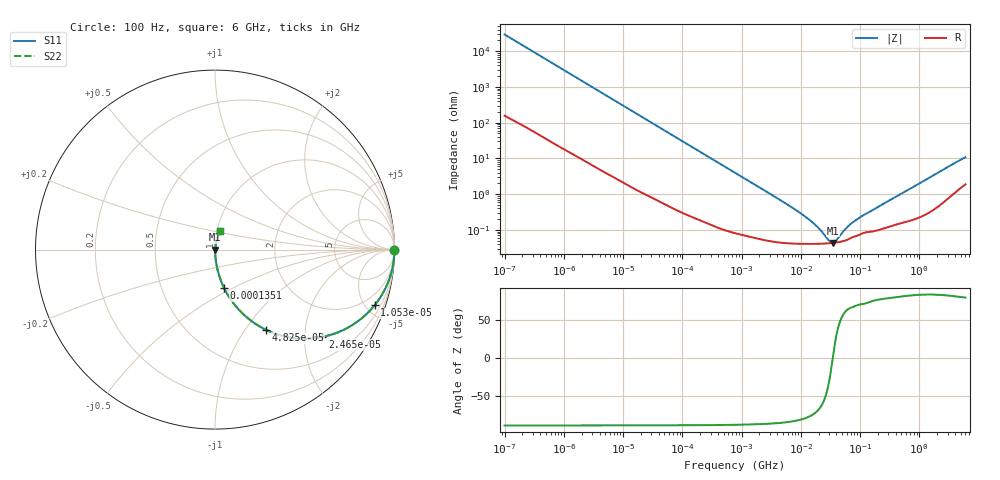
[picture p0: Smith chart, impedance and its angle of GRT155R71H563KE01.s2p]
!Murata Part Number: GRT155R71H563KE01
!These Parameters are Measured in Series Mode Connection
!Data Generated on Jun 19, 2026
!  o--ll--o
!Port1  Port2
!  o------o
!Operation Temp=25[degC], DC Bias Voltage=0[V]
!Freq. Start=100[Hz] Stop=6[GHz] 401[Steps]
# Hz S RI R 50
!Freq.(Hz) S11(Real) S11(Imag) S21(Real) S21(Imag) S12(Real) S12(Imag) S22(Real) S22(Imag)
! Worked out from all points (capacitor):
!   401 points, 100 Hz to 6 GHz, reference 50 ohm
!   read as one part in series: C = 53.9 nF near 109 Hz
!   lowest |Z| = 43.2 mohm at 34.83 MHz (marker M1)
!   series resonance near 34.63 MHz, so ESL is about 390 pH
!   S11 on the Smith chart (normalised r, x): 100 Hz: open; 10.53 kHz: 1.04, -5.70; 24.65 kHz: 1.02, -2.45; 48.25 kHz: 1.01, -1.25; 135.1 kHz: 1.00, -0.45; 6 GHz: 1.04, +0.21
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100  1 -0.00339  2.95e-05 0.00339  2.95e-05 0.00339  1 -0.00339
2008  0.9951 -0.067  0.00493 0.067  0.00493 0.067  0.9951 -0.067
4918  0.9727 -0.1596  0.0273 0.1596  0.0273 0.1596  0.9727 -0.1596
10527  0.8888 -0.3108  0.1112 0.3108  0.1112 0.3108  0.8888 -0.3108
15752  0.7831 -0.4085  0.2169 0.4085  0.2169 0.4085  0.7831 -0.4085
24648  0.5985 -0.4863  0.4015 0.4863  0.4015 0.4863  0.5985 -0.4863
40335  0.3605 -0.476  0.6395 0.476  0.6395 0.476  0.3605 -0.476
48246  0.2837 -0.4465  0.7163 0.4465  0.7163 0.4465  0.2837 -0.4465
78952  0.1308 -0.3325  0.8692 0.3325  0.8692 0.3325  0.1308 -0.3325
135116  0.0502 -0.2132  0.9498 0.2132  0.9498 0.2132  0.0502 -0.2132
289253  0.0124 -0.1041  0.9876 0.1041  0.9876 0.1041  0.0124 -0.1041
774597  0.00237 -0.0395  0.9976 0.0395  0.9976 0.0395  0.00237 -0.0395
6353432  0.000441 -0.00474  0.9996 0.00474  0.9996 0.00474  0.000441 -0.00474
1.555665e7  0.000407 -0.0016  0.9996 0.0016  0.9996 0.0016  0.000407 -0.0016
2.128304e7  0.00041 -0.000912  0.9996 0.000912  0.9996 0.000912  0.00041 -0.000912
3.045065e7  0.000422 -0.000232  0.9996 0.000232  0.9996 0.000232  0.000422 -0.000232
3.482834e7  0.000431 1.07e-05  0.9996 -1.07e-05  0.9996 -1.07e-05  0.000431 1.07e-05
3.983537e7  0.000443 0.000254  0.9996 -0.000254  0.9996 -0.000254  0.000443 0.000254
5.699437e7  0.000507 0.000936  0.9995 -0.000936  0.9995 -0.000936  0.000507 0.000936
7.455971e7  0.000625 0.00148  0.9994 -0.00148  0.9994 -0.00148  0.000625 0.00148
3.124326e8  0.00128 0.00654  0.9987 -0.00654  0.9987 -0.00654  0.00128 0.00654
6e9  0.0289 0.101  0.9711 -0.101  0.9711 -0.101  0.0289 0.101
